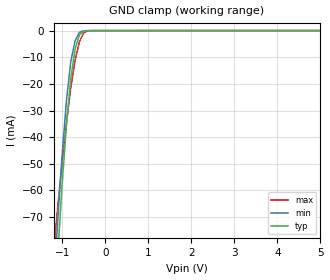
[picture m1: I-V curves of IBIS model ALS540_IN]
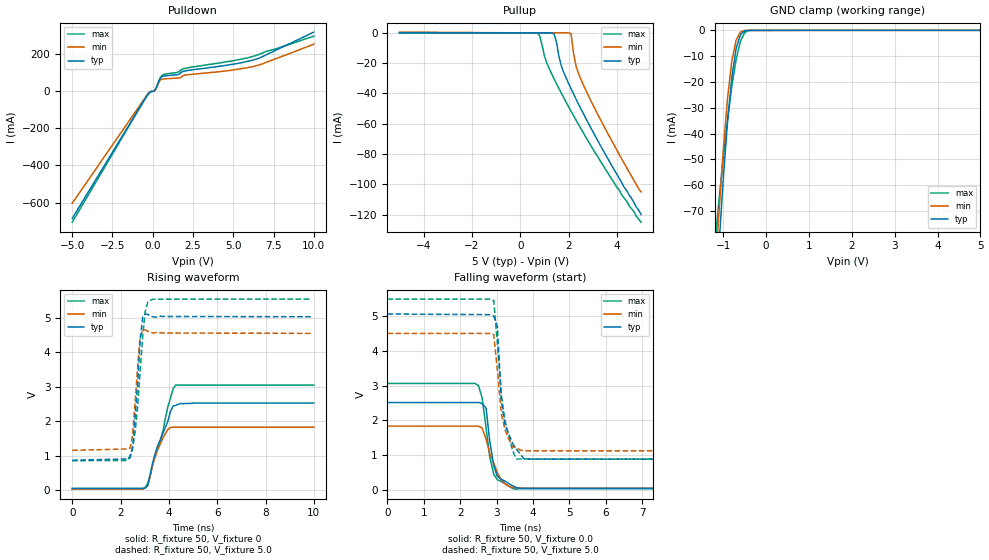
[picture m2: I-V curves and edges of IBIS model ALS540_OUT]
| TEXAS INSTRUMENTS INCORPORATED
| Standard Linear and Logic Group
| IBIS Model of SN74ALS540
| OCTAL BUFFERS AND LINE DRIVERS WITH 3-STATE OUTPUTS
| SOIC 20-pin (DW), SOP 20-pin (NS), SSOP 20-pin (DB), P-DIP 20-pin (N) Package
[IBIS Ver]   3.2
[Comment Char]  |_char
[File Name]   sn74als540.ibs
[File Rev]   2.1
[Date]   Sept. 27, 2004
[Source]   Data created from Lab. data at TI-SLL.
[Notes]   The following is an IBIS list for the ALS540.
   Please contact sllibis@ti.com with questions and
   comments concerning SLL IBIS models.
   - FILE REV HISTORY
   - 2.1 Re-Release IBIS file on 10/06/04
   - Power clamp data deleted as there is no power-clamp diode.
[Disclaimer] Property of Texas Instruments Incorporated.  Unauthorized
   reproduction and/or distribution is strictly prohibited.
   This product is protected under copyright law.
   Created 2000, (C) Copyright 2000, Texas Instruments Inc.,
   All Rights Reserved.
   UNLESS THERE IS A SIGNED, WRITTEN AGREEMENT TO THE
   CONTRARY, TEXAS INSTRUMENTS () IS PROVIDING THE IBIS
   MODELS  AND WITHOUT ANY WARRANTY, EXPRESSED OR
   IMPLIED.  TI assumes no liability for:
   1) the accuracy of the IBIS models provided to your
   company;
   2) the proper functioning of these IBIS Models in your
   design or for any resulting applications; or
   3) infringement of patents, copyrights or intellectual
   property rights resulting from your use of these IBIS
   models.
   TI provides IBIS Models as a service to our customers.
   You and your company shall not distribute, sell or give
   these models to anyone else without prior written
   permission from TI.
   TI reserves the right to make changes to our products or
   to discontinue any semiconductor product or service
   without notice, and advises our customers to obtain the
   latest version of relevant information to verify, before
   placing orders, that the information being relied on is
   current.
   Please be aware that your receipt and use of the IBIS
   information provided shall serve as acceptance of these
   terms and conditions.  If you do not accept these terms,
   you should return or destroy the IBIS models and any
   other accompanying information immediately.
|   Component ALS540_DW
[Component]   ALS540_DW
[Manufacturer]   Texas Instruments, Inc.
[Package]
|   typ   min   max
R_pkg   0.038   0.033   0.045
L_pkg   5.012nH   4.110nH   6.349nH
C_pkg   0.717pF   0.530pF   0.868pF
[Pin]   signal_name   model_name   R_pin   L_pin   C_pin
1   1OE_NOT   ALS540_IN   0.042   6.336nH   0.865pF
2   A1   ALS540_IN   0.043   5.542nH   0.867pF
3   A2   ALS540_IN   0.034   4.714nH   0.732pF
4   A3   ALS540_IN   0.034   4.377nH   0.591pF
5   A4   ALS540_IN   0.036   4.130nH   0.533pF
6   A5   ALS540_IN   0.035   4.111nH   0.530pF
7   A6   ALS540_IN   0.034   4.284nH   0.583pF
8   A7   ALS540_IN   0.034   4.634nH   0.726pF
9   A8   ALS540_IN   0.040   5.518nH   0.865pF
10   GND   GND   0.043   6.349nH   0.866pF
11   Y8   ALS540_OUT   0.041   6.281nH   0.861pF
12   Y7   ALS540_OUT   0.045   5.561nH   0.868pF
13   Y6   ALS540_OUT   0.033   4.778nH   0.742pF
14   Y5   ALS540_OUT   0.035   4.414nH   0.596pF
15   Y4   ALS540_OUT   0.035   4.110nH   0.533pF
16   Y3   ALS540_OUT   0.036   4.130nH   0.533pF
17   Y2   ALS540_OUT   0.034   4.377nH   0.591pF
18   Y1   ALS540_OUT   0.034   4.714nH   0.731pF
19   2OE_NOT   ALS540_OUT   0.043   5.569nH   0.868pF
20   VCC   POWER   0.042   6.308nH   0.864pF
|   Component ALS540_NS
[Component]   ALS540_NS
[Manufacturer]  Texas Instruments, Inc.
[Package]
|   typ   min   max
R_pkg   0.044   0.029   0.058
L_pkg   3.666nH   2.317nH   5.115nH
C_pkg   0.548pF   0.316pF   0.725pF
[Pin]   signal_name   model_name   R_pin   L_pin   C_pin
1   1OE_NOT   ALS540_IN   0.058   5.115nH   0.725pF
2   A1   ALS540_IN   0.053   4.591nH   0.724pF
3   A2   ALS540_IN   0.049   3.754nH   0.572pF
4   A3   ALS540_IN   0.029   2.549nH   0.388pF
5   A4   ALS540_IN   0.031   2.317nH   0.316pF
6   A5   ALS540_IN   0.031   2.317nH   0.316pF
7   A6   ALS540_IN   0.029   2.556nH   0.399pF
8   A7   ALS540_IN   0.049   3.754nH   0.579pF
9   A8   ALS540_IN   0.053   4.591nH   0.724pF
10   GND   GND   0.058   5.115nH   0.725pF
11   Y8   ALS540_OUT   0.058   5.115nH   0.725pF
12   Y7   ALS540_OUT   0.053   4.591nH   0.724pF
13   Y6   ALS540_OUT   0.049   3.754nH   0.579pF
14   Y5   ALS540_OUT   0.029   2.557nH   0.399pF
15   Y4   ALS540_OUT   0.031   2.317nH   0.316pF
16   Y3   ALS540_OUT   0.031   2.317nH   0.316pF
17   Y2   ALS540_OUT   0.029   2.557nH   0.399pF
18   Y1   ALS540_OUT   0.049   3.754nH   0.579pF
19   2OE_NOT   ALS540_OUT   0.053   4.591nH   0.724pF
20   VCC   POWER   0.058   5.115nH   0.725pF
|   Component ALS540_DB
[Component]   ALS540_DB
[Manufacturer]   Texas Instruments, Inc.
[Package]
|   typ   min   max
R_pkg   0.040   0.035   0.051
L_pkg   3.495nH   3.035nH   4.314nH
C_pkg   0.420pF   0.346pF   0.502pF
[Pin]   signal_name   model_name   R_pin   L_pin   C_pin
1   1OE_NOT   ALS540_IN   0.049   4.310nH   0.502pF
2   A1   ALS540_IN   0.048   3.903nH   0.487pF
3   A2   ALS540_IN   0.035   3.189nH   0.396pF
4   A3   ALS540_IN   0.035   3.036nH   0.347pF
5   A4   ALS540_IN   0.035   3.035nH   0.367pF
6   A5   ALS540_IN   0.035   3.035nH   0.367pF
7   A6   ALS540_IN   0.035   3.036nH   0.347pF
8   A7   ALS540_IN   0.035   3.189nH   0.397pF
9   A8   ALS540_IN   0.047   3.899nH   0.488pF
10   GND   GND   0.051   4.314nH   0.500pF
11   Y8   ALS540_OUT   0.051   4.314nH   0.500pF
12   Y7   ALS540_OUT   0.047   3.899nH   0.488pF
13   Y6   ALS540_OUT   0.035   3.189nH   0.397pF
14   Y5   ALS540_OUT   0.035   3.036nH   0.346pF
15   Y4   ALS540_OUT   0.035   3.035nH   0.367pF
16   Y3   ALS540_OUT   0.035   3.035nH   0.367pF
17   Y2   ALS540_OUT   0.035   3.036nH   0.346pF
18   Y1   ALS540_OUT   0.035   3.189nH   0.397pF
19   2OE_NOT   ALS540_OUT   0.047   3.899nH   0.488pF
20   VCC   POWER   0.051   4.314nH   0.502pF
|   Component ALS540_N
[Component]   ALS540_N
[Manufacturer]  Texas Instruments, Inc.
[Package]
|   Mean.   Min.   Max.
R_pkg   0.043   0.038   0.05
L_pkg   7.384nH   4.68nH   10.321nH
C_pkg   0.51pF   0.231pF   0.821pF
[Pin]   signal_name   model_name   R_pin   L_pin   C_pin
1   1OE_NOT   ALS540_IN   0.042   9.427nH   0.81pF
2   A1   ALS540_IN   0.046   8.544nH   0.456pF
3   A2   ALS540_IN   0.048   7.163nH   0.435pF
4   A3   ALS540_IN   0.04   4.825nH   0.261pF
5   A4   ALS540_IN   0.04   5.284nH   0.648pF
6   A5   ALS540_IN   0.04   4.686nH   0.232pF
7   A6   ALS540_IN   0.04   6.359nH   0.489pF
8   A7   ALS540_IN   0.038   7.982nH   0.475pF
9   A8   ALS540_IN   0.043   9.403nH   0.475pF
10   GND   GND   0.05   10.321nH  0.805pF
11   Y8   ALS540_OUT   0.05   10.281nH  0.81pF
12   Y7   ALS540_OUT   0.043   9.383nH   0.477pF
13   Y6   ALS540_OUT   0.038   7.978nH   0.476pF
14   Y5   ALS540_OUT   0.04   6.302nH   0.492pF
15   Y4   ALS540_OUT   0.04   4.68nH   0.231pF
16   Y3   ALS540_OUT   0.04   5.284nH   0.648pF
17   Y2   ALS540_OUT   0.04   4.822nH   0.261pF
18   Y1   ALS540_OUT   0.047   7.118nH   0.439pF
19   2OE_NOT   ALS540_OUT   0.046   8.492nH   0.461pF
20   VCC   POWER   0.043   9.348nH   0.821pF
| Models and submodels in the file (2): ALS540_IN (Input), ALS540_OUT (3-state)
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|   Model ALS540_IN
[Model]   ALS540_IN
Model_type  Input
Polarity   Inverting
Vinl = 0.8
Vinh = 2.0
| variable   typ   min   max
C_comp   1.33pf   1.00pf   1.66pf
[Temperature Range]   25   0   70
[Voltage Range]   5.0   4.5   5.5
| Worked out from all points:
|   GND clamp passes 1 mA (typ) near -0.56 V on its own axis
[GND Clamp]
|   Voltage   I(typ)   I(min)   I(max)
-5V       -1.31A     -1.3A      -904mA
-1.2V     -112mA     -97.6mA    -83.8mA
-1.1V     -83.5mA    -70.6mA    -65.8mA
-1V       -57.7mA    -46.6mA    -49.3mA
-900mV    -35.4mA    -26.3mA    -34.6mA
-800mV    -18.2mA    -11.8mA    -21.6mA
-700mV    -6.99mA    -3.84mA    -11.3mA
-600mV    -1.67mA    -654uA     -4.26mA
-500mV    -155uA     -44.6uA    -872uA
-400mV    -25.2uA    -22.8uA    -77.5uA
5V        220pA      78.9pA     2.28nA
|   Model ALS540_OUT
[Model]   ALS540_OUT
Model_type  3-state
Polarity   Non-Inverting
Enable   Active-Low
Vmeas = 2.5v
Cref = 15pf
| variable   typ   min   max
C_comp   5.8pf   4.35pf   7.25pf
[Temperature Range]   25   0   70
[Voltage Range]   5.0   4.5   5.5
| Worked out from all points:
|   slope of the pulldown table from 0 to 0.75 V, typ, clamps not added: 9.1 ohm
|   GND clamp passes 1 mA (typ) near -0.56 V on its own axis
|   rising waveform, R_fixture 50, V_fixture 0: 20-80 % time 718ps typ, 503ps min, 670ps max; typ from 0.06 V to 2.53 V
|   falling waveform, R_fixture 50, V_fixture 0.0: 20-80 % time 228ps typ, 360ps min, 254ps max; typ from 2.51 V to 0.033 V
|   rising waveform, R_fixture 50, V_fixture 5.0: 20-80 % time 247ps typ, 217ps min, 320ps max; typ from 0.873 V to 5.03 V
|   falling waveform, R_fixture 50, V_fixture 5.0: 20-80 % time 243ps typ, 232ps min, 281ps max; typ from 5.06 V to 0.88 V
[Pulldown]
|   Voltage   I(typ)   I(min)   I(max)
-5V       -685mA     -603mA     -705mA
-300mV    -17.3mA    -13.6mA    -19.8mA
-100mV    -2.38mA    -1.65mA    -3.44mA
100mV     1.24mA     60.3uA     2.33mA
200mV     14.6mA     10.8mA     15.8mA
400mV     58.2mA     50.8mA     57.2mA
600mV     78.9mA     64.4mA     86mA
1.6V      89.2mA     70mA       103mA
2.1V      110mA      87mA       124mA
5V        144mA      114mA      163mA
6.4V      171mA      136mA      191mA
10V       317mA      252mA      295mA
[Pullup]
|   Voltage   I(typ)   I(min)   I(max)
-5V       19.3nA     497uA      2.13nA
700mV     19.3nA     299nA      -120uA
800mV     19.3nA     252nA      -1.83mA
1V        19.3nA     95.8nA     -15.4mA
1.4V      -819uA     60.3nA     -30.4mA
1.7V      -21.9mA    42.9nA     -39.8mA
2.1V      -36.9mA    -454uA     -51.7mA
2.2V      -40.2mA    -13.2mA    -54.6mA
2.3V      -43.5mA    -21.4mA    -57.4mA
2.6V      -53mA      -34mA      -65.7mA
3.7V      -85.2mA    -68.8mA    -94.4mA
5V        -120mA     -105mA     -125mA
[GND Clamp]
|   Voltage   I(typ)   I(min)   I(max)
-5V       -1.31A     -1.3A      -904mA
-1.2V     -112mA     -97.6mA    -83.8mA
-1.1V     -83.5mA    -70.6mA    -65.8mA
-1V       -57.7mA    -46.6mA    -49.3mA
-900mV    -35.4mA    -26.3mA    -34.6mA
-800mV    -18.2mA    -11.8mA    -21.6mA
-700mV    -6.99mA    -3.84mA    -11.3mA
-600mV    -1.67mA    -654uA     -4.26mA
-500mV    -155uA     -44.6uA    -872uA
-400mV    -25.2uA    -22.8uA    -77.5uA
5V        220pA      78.9pA     2.28nA
[Ramp]
| variable   typ   min   max
dV/dt_r   1.49E+00/6.83E-10   1.27E+00/6.73E-09   1.67E+00/6.02E-10
dV/dt_f   2.57E+00/2.72E-10   2.05E+00/1.89E-09   2.81E+00/2.83E-10
R_load = 50
[Rising Waveform]
R_fixture = 50
V_fixture = 0
|   Time   V(typ)   V(min)   V(max)
0s        60.4mV     44.3mV     35.5mV
3.02ns    65.5mV     69.7mV     83.8mV
3.13ns    155mV      137mV      216mV
3.33ns    807mV      745mV      737mV
3.44ns    1.08V      982mV      1.02V
3.75ns    1.65V      1.52V      1.7V
3.96ns    2.01V      1.77V      2.43V
4.17ns    2.44V      1.83V      2.93V
4.27ns    2.46V      1.83V      3.05V
10ns      2.53V      1.83V      3.05V
[Falling Waveform]
R_fixture = 50
V_fixture = 0.0
|   Time   V(typ)   V(min)   V(max)
0s        2.51V      1.83V      3.06V
2.5ns     2.51V      1.83V      3V
2.6ns     2.48V      1.78V      2.65V
2.71ns    2.35V      1.46V      1.78V
2.81ns    1.4V       1.04V      946mV
2.92ns    696mV      768mV      449mV
3.02ns    383mV      485mV      283mV
3.13ns    299mV      276mV      235mV
3.44ns    112mV      69mV       34mV
10ns      32.6mV     39.9mV     30.2mV
[Rising Waveform]
R_fixture = 50
V_fixture = 5.0
V_fixture_min = 4.5
V_fixture_max = 5.5
|   Time   V(typ)   V(min)   V(max)
0s        873mV      1.16V      862mV
2.4ns     945mV      1.23V      1.02V
2.5ns     1.28V      1.61V      1.21V
2.6ns     2.11V      2.54V      1.68V
2.71ns    3.15V      3.6V       2.45V
2.81ns    4.34V      4.45V      3.46V
2.92ns    5.03V      4.65V      4.49V
3.02ns    5.11V      4.65V      5.19V
3.13ns    5.1V       4.61V      5.46V
9.9ns     5.03V      4.55V      5.544V
[Falling Waveform]
R_fixture = 50
V_fixture = 5.0
V_fixture_min = 4.5
V_fixture_max = 5.5
|   Time   V(typ)   V(min)   V(max)
0s        5.06V      4.5V       5.49V
2.92ns    5V         4.47V      5.45V
3.02ns    4.7V       3.45V      4.24V
3.13ns    2.56V      2.19V      2.73V
3.23ns    1.86V      1.73V      1.99V
3.44ns    1.33V      1.23V      1.12V
3.54ns    1.17V      1.21V      884mV
3.75ns    888mV      1.12V      884mV
3.85ns    880mV      1.12V      886mV
10ns      880mV      1.12V      881mV
